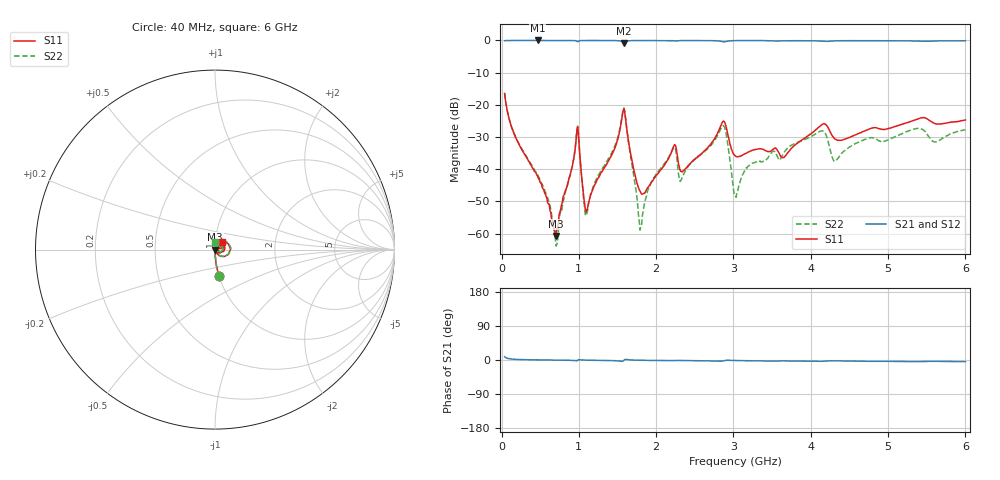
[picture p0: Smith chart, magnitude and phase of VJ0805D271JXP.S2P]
! VJ0805D271JXP
! DATE 03/14/2022  09:16
! CAPACITORS MOUNTED IN SERIES ON 25 MIL THICK MICROSTRIP SUBSTRATE
# GHz  S  MA  R  50.00
!  FREQ  S11M  S11A  S21M  S21A  S12M  S12A  S22M  S22A
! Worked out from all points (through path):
!   600 points, 40 MHz to 6 GHz, reference 50 ohm
!   highest |S21| = 0.00 dB at 467.9 MHz (marker M1); lowest = -0.8 dB at 1.582 GHz (marker M2)
!   lowest |S11| = -60.7 dB at 706.6 MHz (marker M3), VSWR 1.00, Z = 50.1 + j0.0244 ohm
!   |S11| at or under -10 dB: start of sweep to end of sweep
!   |S22| runs from -63.9 to -16.4 dB; largest |S21 - S12| = 0.0033
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0.04  0.1499 -81.4  0.9884 8.6  0.987 8.6  0.1511 -81.7
0.16935  0.03385 -87.7  0.999 1.9  0.9995 1.9  0.03426 -87.8
0.46785  0.007758 -86.2  0.9999 0.2  1 0.3  0.008273 -86.7
0.70665  0.0009184 15.4  0.9995 -0.3  1 -0.3  0.0006361 -3.6
0.96535  0.02918 53.0  0.9837 -1.8  0.9847 -1.8  0.02997 57.3
0.9952  0.03362 -34.9  0.9716 0.7  0.9722 0.6  0.03454 -31.6
1.035  0.007964 -58.1  0.9962 -0.0  0.9968 -0.1  0.008099 -56.1
1.10465  0.002339 20.0  0.9983 -0.5  0.9986 -0.5  0.002068 31.8
1.58225  0.08679 1.9  0.9125 -1.1  0.9132 -1.1  0.08944 5.4
1.7912  0.004559 -23.5  0.9972 -0.7  0.9981 -0.7  0.001132 -11.8
2.03  0.008811 51.7  0.9973 -1.3  0.9988 -1.4  0.009295 88.9
2.229  0.02306 36.1  0.9863 -1.9  0.9871 -2.0  0.02191 59.8
2.3285  0.009177 21.9  0.9952 -1.3  0.9961 -1.3  0.006981 68.9
2.8658  0.05537 17.4  0.9562 -2.6  0.9569 -2.6  0.04759 31.8
3.025  0.01607 -5.0  0.9936 -1.3  0.995 -1.4  0.003769 28.9
3.21405  0.01896 21.2  0.9976 -2.1  0.9974 -2.0  0.01155 84.7
3.6419  0.0151 32.2  0.9859 -2.4  0.987 -2.4  0.01727 102.1
4.02  0.03695 48.0  0.9881 -3.2  0.9894 -3.3  0.03286 84.0
4.16925  0.05076 27.4  0.968 -3.3  0.9696 -3.3  0.03854 53.3
4.3185  0.02918 16.3  0.9855 -2.2  0.9859 -2.3  0.01332 66.9
5.015  0.04304 40.7  0.9898 -3.5  0.9906 -3.6  0.02888 93.1
6.00005  0.05822 46.1  0.9881 -4.4  0.9891 -4.5  0.04097 92.1
